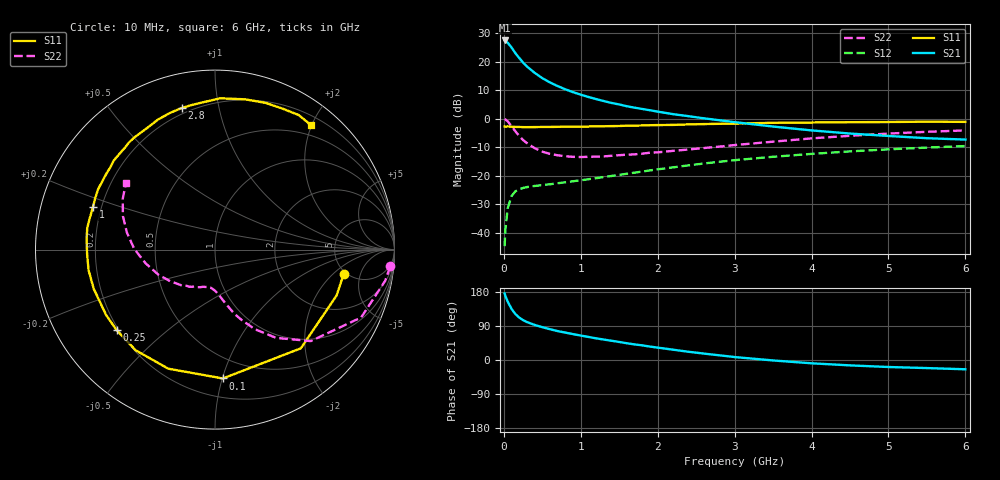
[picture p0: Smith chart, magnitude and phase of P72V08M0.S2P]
! SIEMENS Small Signal Semiconductors
! BFP196
! Si NPN RF Bipolar Junction Transistor in SOT143
! VCE = 2 V  IC = 8 mA
! Common Emitter S-Parameters:  May  1996
# GHz  S  MA  R  50
!  f  S11  S21  S12  S22
! GHz  MAG  ANG  MAG  ANG  MAG  ANG  MAG  ANG
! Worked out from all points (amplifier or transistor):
!   36 points, 10 MHz to 6 GHz, reference 50 ohm
!   highest |S21| = 27.4 dB at 10 MHz (marker M1)
!   |S21| within 3 dB of that: start of sweep to 113.2 MHz
!   unconditionally stable (mu >= 1): 929.2 MHz to 3.304 GHz; 5.963 GHz to end of sweep
!   at 250 MHz: K = 0.35, MSG = 22.0 dB, |S12| = -24.3 dB
!   at 1.4 GHz: K = 1.16, MAG = 10.4 dB, |S12| = -20.1 dB
!   at 6 GHz: K = 1.00, MAG = 0.8 dB, |S12| = -9.6 dB
!   S11 on the Smith chart (normalised r, x): 10 MHz: 4.75, -2.75; 100 MHz: 0.34, -1.00; 250 MHz: 0.19, -0.35; 1 GHz: 0.17, +0.16; 2.8 GHz: 0.17, +0.78; 6 GHz: 0.33, +1.98
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0.01  0.7298 -10.7  23.44 175.5  0.0058 84.9  0.9805 -5.5
0.02  0.7241 -20.7  22.77 169.0  0.0112 80.5  0.964 -10.4
0.05  0.7288 -49.0  21.41 154.3  0.0268 66.3  0.8979 -24.9
0.1  0.7193 -86.5  17.62 134.8  0.0438 51.2  0.7378 -43.7
0.15  0.7127 -111.4  14.03 121.2  0.0532 41.7  0.5983 -55.3
0.2  0.7141 -128.2  11.57 112.0  0.0577 36.0  0.4961 -63.4
0.25  0.7086 -140.6  9.594 105.2  0.0608 32.5  0.4204 -69.2
0.3  0.7077 -149.1  8.197 100.2  0.063 30.5  0.3725 -73.3
0.4  0.7101 -162.1  6.353 92.6  0.0659 29.1  0.303 -79.2
0.5  0.7137 -170.8  5.115 86.6  0.0682 29.1  0.263 -83.8
0.6  0.713 -178.0  4.297 81.2  0.0707 29.9  0.2405 -87.4
0.7  0.7175 175.5  3.715 76.3  0.0736 31.1  0.2273 -90.6
0.8  0.722 170.5  3.259 72.3  0.0765 31.9  0.2189 -93.7
1  0.7199 160.9  2.622 64.5  0.0828 35.1  0.2122 -99.5
1.1  0.7264 156.8  2.392 60.8  0.0864 36.3  0.2134 -102.5
1.6  0.7514 138.6  1.646 44.2  0.108 40.1  0.233 -116.3
2.2  0.775 119.6  1.197 27.2  0.1398 40.8  0.2721 -132.6
2.8  0.8105 103.2  0.936 12.4  0.1749 37.4  0.3224 -150.4
3.5  0.8436 88.0  0.725 -1.2  0.2141 30.7  0.394 -168.8
4.5  0.8648 70.9  0.547 -14.2  0.2662 19.7  0.4996 169.1
5.5  0.8829 58.1  0.453 -21.3  0.3105 8.1  0.5869 151.1
6  0.876 52.5  0.429 -24.5  0.3303 1.8  0.6211 143.0
